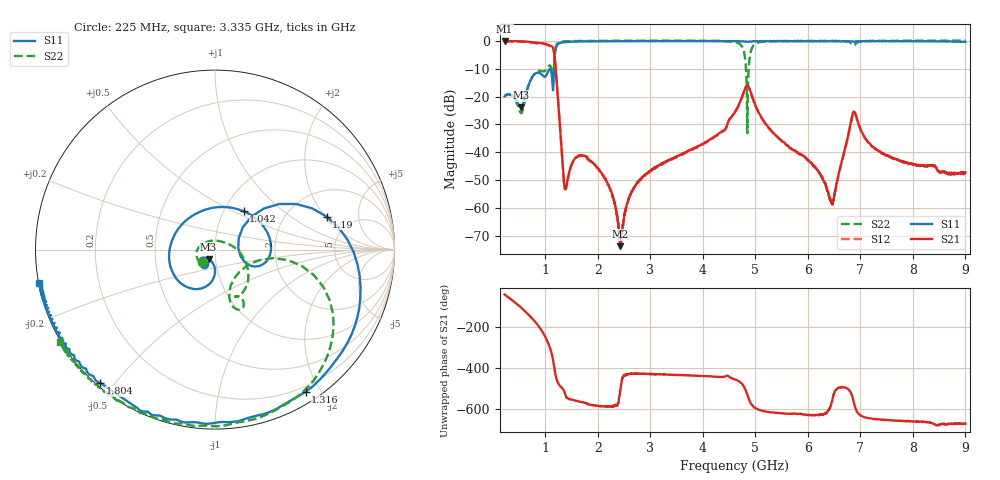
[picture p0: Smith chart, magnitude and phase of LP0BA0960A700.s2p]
!Agilent Technologies,E8358A,US41080443,A.07.50.56
!Agilent E8358A: A.07.50.56
!Date: Wednesday, August 31, 2016 09:19:48
!Correction: S11(Full 2 Port(1,2))
!S21(Full 2 Port(1,2))
!S12(Full 2 Port(1,2))
!S22(Full 2 Port(1,2))
!S2P File: Measurements: S11, S21, S12, S22:
# Hz S  dB  R 50
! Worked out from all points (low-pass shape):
!   1601 points, 225 MHz to 9 GHz, reference 50 ohm
!   highest |S21| = -0.04 dB at 225 MHz (marker M1); lowest = -73.8 dB at 2.424 GHz (marker M2)
!   |S21| within 3 dB of the highest: start of sweep to 1.157 GHz
!   lowest |S11| = -23.8 dB at 532.1 MHz (marker M3), VSWR 1.14, Z = 46.3 - j4.98 ohm
!   |S11| at or under -10 dB: start of sweep to 1.166 GHz
!   |S22| runs from -33.2 to 0.2 dB; largest |S21 - S12| = 0.022
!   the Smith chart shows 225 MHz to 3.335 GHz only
!   S11 on the Smith chart (normalised r, x): 225 MHz: 0.87, -0.14; 1.042 GHz: 1.24, +0.57; 1.19 GHz: 3.28, +2.09; 1.316 GHz: 0.14, -1.82; 1.804 GHz: 0.01, -0.46; 3.335 GHz: 0.00, -0.09
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2.25e8  -19.93 -127.9  -0.04 -42.2  -0.22 -41.9  -19.80 -136.4
5.32125e8  -23.84 -123.6  -0.12 -104.1  -0.31 -104.0  -25.88 98.6
8.337656e8  -11.49 -133.6  -0.66 177.0  -0.85 177.2  -11.11 -53.9
1.042172e9  -11.49 53.1  -1.30 88.6  -1.46 88.9  -9.59 -61.5
1.124438e9  -12.36 -23.1  -1.96 27.5  -2.15 27.7  -11.09 -73.4
1.19025e9  -3.76 16.5  -8.09 -66.7  -8.27 -66.6  -3.09 -24.0
1.316391e9  -0.55 -57.5  -40.58 -135.6  -40.80 -135.4  -0.27 -78.5
1.393172e9  -0.41 -75.9  -53.05 -177.1  -53.02 -177.7  -0.15 -91.7
1.689328e9  -0.15 -110.2  -41.10 155.6  -41.31 155.4  -0.00 -118.7
1.8045e9  -0.18 -130.7  -42.43 144.8  -42.57 145.0  -0.02 -122.3
2.424234e9  -0.08 -155.2  -73.77 -149.1  -71.41 -174.8  0.05 -139.0
3.153656e9  -0.10 -167.1  -44.90 -69.5  -45.02 -69.1  0.02 -147.1
3.334641e9  -0.02 -169.2  -42.98 -71.8  -43.24 -71.3  0.06 -149.2
4.6125e9  -0.12 -178.0  -25.55 -94.6  -25.72 -94.3  -0.40 -174.6
4.788e9  -0.25 179.4  -17.89 -132.6  -18.07 -131.9  -4.39 149.1
4.864781e9  -0.35 -180.0  -16.36 177.2  -16.50 177.4  -13.19 -87.9
5.133516e9  -0.14 178.1  -28.09 112.9  -28.27 113.5  -0.33 -148.2
6.076828e9  -0.04 166.2  -43.88 91.8  -44.24 92.0  0.02 -176.3
6.466219e9  -0.04 160.9  -58.88 167.8  -57.86 169.0  0.03 175.3
6.883031e9  -0.32 155.7  -25.46 146.2  -25.63 146.4  -1.57 171.1
7.541156e9  -0.18 148.5  -41.32 67.3  -41.61 67.8  -0.01 160.7
9e9  -0.35 129.3  -47.28 49.3  -47.73 47.8  0.14 150.6
